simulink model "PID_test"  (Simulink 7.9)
settings: Solver=ode45  StartTime=0.0  StopTime=10.0  RelTol=1e-3
libraries: EMG30 x1

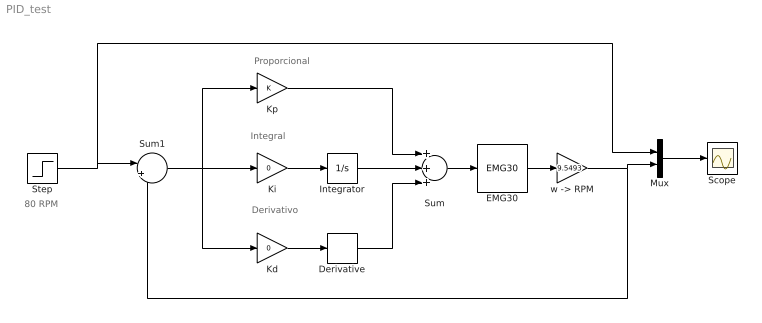
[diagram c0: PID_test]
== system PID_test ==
  note: Proporcional
  note: Integral
  note: Derivativo
  note: 80 RPM
  Derivative : Derivative
  EMG30 : EMG30/EMG30  R=7.101  L=0.0034  J=0.0019  b=0.000931  Kt=0.509  Ke=0.509  Tc=0.04
  Integrator : Integrator
  Kd : Gain  Gain=0
  Ki : Gain  Gain=0
  Kp : Gain
  Mux : Mux  Inputs=2
  Scope : Scope
  Step : Step  After=80  SampleTime=0
  Sum : Sum  Inputs=+++
  Sum1 : Sum  Inputs=|+-
  "w -> RPM" : Gain  Gain=9.5493
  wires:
  Ki/1 -> Integrator/1
  Kp/1 -> Sum/1
  Integrator/1 -> Sum/2
  Derivative/1 -> Sum/3
  Kd/1 -> Derivative/1
  Sum/1 -> EMG30/1
  Sum1/1 -> Kd/1, Ki/1, Kp/1
  Step/1 -> Sum1/1, Mux/1
  Mux/1 -> Scope/1
  EMG30/1 -> "w -> RPM"/1
  "w -> RPM"/1 -> Mux/2, Sum1/2
